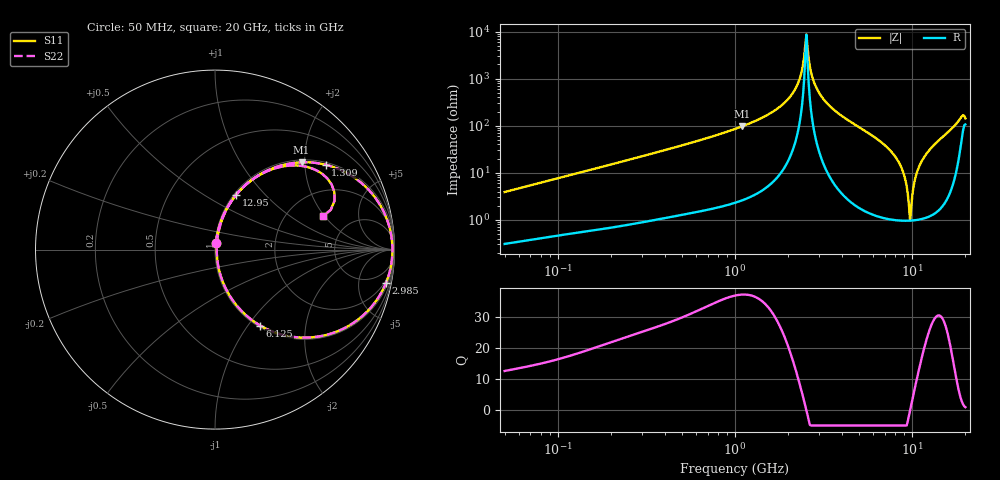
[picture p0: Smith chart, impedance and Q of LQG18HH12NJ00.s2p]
!Murata Part Number: LQG18HH12NJ00
!These Parameters are Measured in Series Mode Connection
!  o--[Z]--o
!Port1  Port2
!  o-------o
!Freq. Start=50[MHz] Stop=20[GHz], 401[Steps]
# Hz S RI R 50
!Freq.(Hz) S11(Real) S11(Imag) S21(Real) S21(Imag) S12(Real) S12(Imag) S22(Real) S22(Imag)
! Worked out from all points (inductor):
!   401 points, 50 MHz to 20 GHz, reference 50 ohm
!   read as one part in series: L = 12.3 nH near 51.52 MHz
!   highest Q = 37.3 at 1.094 GHz (marker M1), where L = 14 nH
!   self-resonance near 2.494 GHz
!   S11 on the Smith chart (normalised r, x): 50 MHz: 1.01, +0.08; 1.309 GHz: 1.07, +2.55; 2.985 GHz: 2, -10; 6.125 GHz: 1.02, -1.14; 12.95 GHz: 1.03, +0.70; 20 GHz: 3.12, +1.92
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5e7  0.00456 0.0386  0.9954 -0.0386  0.9954 -0.0386  0.00456 0.0386
1.364002e8  0.0158 0.1008  0.9842 -0.1008  0.9842 -0.1008  0.0158 0.1008
3.721004e8  0.0808 0.2547  0.9192 -0.2547  0.9192 -0.2547  0.0808 0.2547
1e9  0.4227 0.4807  0.5773 -0.4807  0.5773 -0.4807  0.4227 0.4807
1.094034e9  0.4826 0.4865  0.5174 -0.4865  0.5174 -0.4865  0.4826 0.4865
1.309461e9  0.616 0.4729  0.384 -0.4729  0.384 -0.4729  0.616 0.4729
1.714689e9  0.8245 0.3637  0.1755 -0.3637  0.1755 -0.3637  0.8245 0.3637
2.083303e9  0.9421 0.2066  0.0579 -0.2066  0.0579 -0.2066  0.9421 0.2066
2.313601e9  0.9783 0.0988  0.0217 -0.0988  0.0217 -0.0988  0.9783 0.0988
2.456456e9  0.9875 0.0324  0.0125 -0.0324  0.0125 -0.0324  0.9875 0.0324
2.531158e9  0.9887 -0.00161  0.0113 0.00161  0.0113 0.00161  0.9887 -0.00161
2.728004e9  0.9811 -0.0874  0.0189 0.0874  0.0189 0.0874  0.9811 -0.0874
2.98453e9  0.9517 -0.1881  0.0483 0.1881  0.0483 0.1881  0.9517 -0.1881
3.908127e9  0.7448 -0.4245  0.2552 0.4245  0.2552 0.4245  0.7448 -0.4245
6.125241e9  0.2516 -0.4232  0.7484 0.4232  0.7484 0.4232  0.2516 -0.4232
7.442007e9  0.0959 -0.2785  0.9041 0.2785  0.9041 0.2785  0.0959 -0.2785
8.774992e9  0.0231 -0.1152  0.9769 0.1152  0.9769 0.1152  0.0231 -0.1152
9.745021e9  0.00953 -0.0007  0.9905 0.0007  0.9905 0.0007  0.00953 -0.0007
1.082228e10  0.0238 0.1162  0.9762 -0.1162  0.9762 -0.1162  0.0238 0.1162
1.295331e10  0.1183 0.3056  0.8817 -0.3056  0.8817 -0.3056  0.1183 0.3056
1.721783e10  0.4818 0.4664  0.5182 -0.4664  0.5182 -0.4664  0.4818 0.4664
2e10  0.6016 0.1856  0.3984 -0.1856  0.3984 -0.1856  0.6016 0.1856
